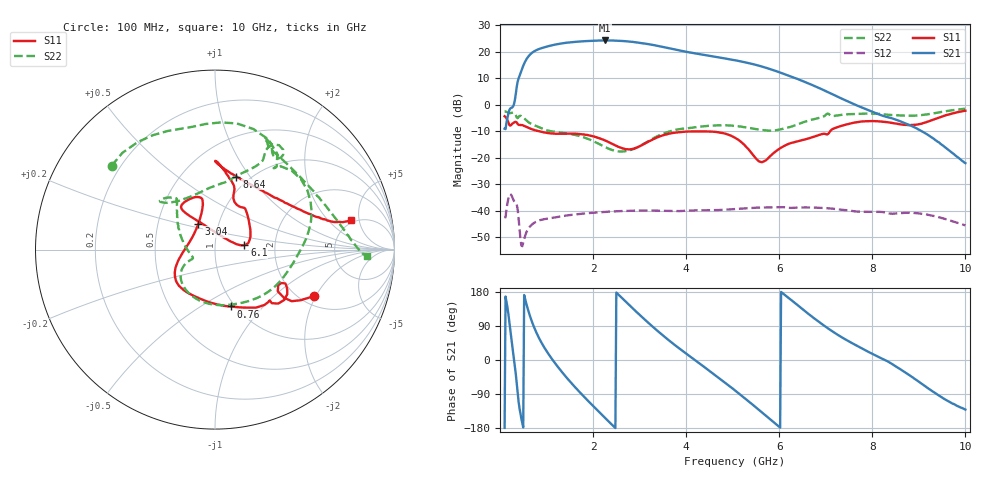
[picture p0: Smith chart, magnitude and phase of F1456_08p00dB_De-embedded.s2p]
! Integrated Device Technology
! Corporate Headquarters
! 6024 Silver Creek Valley Road
! San Jose, CA 95138  USA
! Phone:  1-408-284-8200
! Toll Free:  1-800-223-1366
! Webpage:  http://www.idt.com/
! Timing and RF Division
! 515 Groton Road, Suite 102
! Westford, MA 01886-6024
! Device:  F1456
! Description: 6-bit 0.5 dB Transmit Variable Gain Amplifier
! Frequency:  2100.0 -  2950.00 MHz
! Package:  6x6 mm Thin QFN Plastic Package: 28 pin
! State:  16
! Atten State:  8.0 dB
! Voltage:  +5.00 Volts
! Current:  217.045 mA
! Data:  The device was measured on a the F1455 evaluation board which has
!  individual transmission lines to the RF pins.  Data was collected
!  using a calibrated network analyzer.  The evaluation board was
!  de-embedded using a TRL calibration technique.
!  The reference plane is the edge of the package pin.
!  Pin  1 = CSb
!  Pin  2 = DATA
!  Pin  3 = CLK
!  Pin  4 = RSET
!  Pin  5 = GND
!  Pin  6 = RFIN  = Port 1
!  Pin  7 = GND
!  Pin  8 = NC
!  Pin  9 = NC
!  Pin 10 = NC
!  Pin 11 = NC
!  Pin 12 = NC
!  Pin 13 = NC
!  Pin 14 = /STBY
!  Pin 15 = GND
!  Pin 16 = RFOUT  = Port 2
!  Pin 17 = GND
!  Pin 18 = NC
!  Pin 19 = NC
!  Pin 20 = NC
!  Pin 21 = GND
!  Pin 22 = NC
!  Pin 23 = GND
!  Pin 24 = NC
!  Pin 25 = NC
!  Pin 26 = NC
!  Pin 27 = GND
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# GHz S dB R 50
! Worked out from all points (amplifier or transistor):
!   496 points, 100 MHz to 10 GHz, reference 50 ohm
!   highest |S21| = 24.3 dB at 2.26 GHz (marker M1)
!   |S21| within 3 dB of that: 876.1 MHz to 3.652 GHz (2.776 GHz wide, 123 % of centre)
!   unconditionally stable (mu >= 1): start of sweep to end of sweep
!   at 1.74 GHz: K = 3.27, MAG = 24.5 dB, |S12| = -41.2 dB
!   at 5.06 GHz: K = 5.43, MAG = 17.7 dB, |S12| = -39.3 dB
!   at 10 GHz: K = 136.85, MAG = -12.6 dB, |S12| = -45.5 dB
!   S11 on the Smith chart (normalised r, x): 100 MHz: 2.33, -1.92; 760 MHz: 0.96, -0.68; 3.04 GHz: 0.80, +0.24; 6.1 GHz: 1.39, +0.07; 8.64 GHz: 0.87, +0.86; 10 GHz: 4.62, +3.81
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0.1  -4.33 -25.3  -9.02 -179.2  -42.32 45.1  -2.60 141.0
0.32  -6.50 -31.7  1.73 -16.3  -36.79 -135.0  -3.32 64.1
0.42  -7.62 -42.8  10.89 -127.2  -46.70 139.3  -4.25 45.9
0.58  -8.41 -58.7  17.50 142.6  -47.70 178.8  -6.11 3.6
0.76  -9.65 -74.1  20.43 78.6  -44.30 131.9  -7.88 -25.7
0.98  -10.51 -93.8  21.85 27.7  -43.07 90.6  -9.47 -60.4
1.2  -10.94 -110.9  22.78 -11.1  -42.47 65.2  -10.24 -89.5
1.5  -10.91 -129.1  23.57 -56.1  -41.63 39.2  -10.97 -121.3
1.76  -11.11 -141.4  23.95 -90.9  -41.13 21.0  -12.06 -139.8
2.26  -13.50 -164.0  24.29 -153.0  -40.44 -8.6  -15.95 -156.5
2.62  -16.39 167.9  24.11 163.7  -40.12 -28.3  -17.66 -160.6
3.04  -15.36 122.9  23.32 114.7  -39.94 -50.0  -15.21 170.1
3.4  -12.18 106.4  22.21 75.3  -40.00 -67.7  -11.73 143.2
3.74  -10.59 104.7  20.96 41.2  -40.13 -82.2  -9.59 129.6
4.1  -10.06 112.6  19.70 8.0  -39.96 -96.7  -8.70 128.3
5.06  -12.55 127.1  16.78 -81.2  -39.35 -137.4  -7.98 138.5
5.6  -21.56 64.4  14.58 -135.4  -38.79 -165.4  -9.47 125.1
6.1  -15.60 8.9  11.64 173.5  -38.65 164.8  -8.97 89.9
6.7  -12.34 37.9  7.53 114.8  -38.78 130.5  -5.62 63.6
8.36  -6.67 85.7  -4.80 -5.7  -41.02 56.7  -3.80 62.5
8.64  -7.45 73.6  -6.50 -27.4  -40.83 49.6  -4.06 54.1
10  -2.22 12.3  -22.02 -130.8  -45.52 -28.8  -1.46 -2.5
